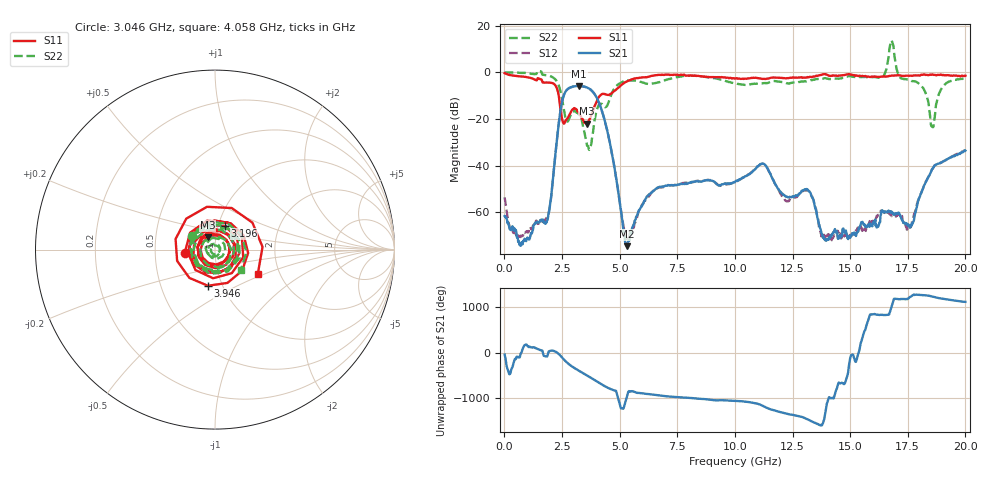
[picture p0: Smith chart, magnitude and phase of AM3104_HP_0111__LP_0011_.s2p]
!Created with skrf (http://scikit-rf.org).
# Hz S RI R 50.0
!freq ReS11 ImS11 ReS21 ImS21 ReS12 ImS12 ReS22 ImS22
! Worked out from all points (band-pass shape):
!   1601 points, 10 MHz to 20 GHz, reference 50 ohm
!   highest |S21| = -5.81 dB at 3.246 GHz (marker M1); lowest = -74.5 dB at 5.332 GHz (marker M2)
!   |S21| within 3 dB of the highest: 2.622 GHz to 3.878 GHz (1.256 GHz wide, 38.6 % of centre)
!   lowest |S11| = -22.1 dB at 3.571 GHz (marker M3), VSWR 1.17, Z = 45.7 + j6.24 ohm
!   |S11| at or under -10 dB: 2.358 GHz to 4.148 GHz (1.79 GHz wide, 55 % of centre)
!   |S22| runs from -33.3 to 13.7 dB; largest |S21 - S12| = 0.027
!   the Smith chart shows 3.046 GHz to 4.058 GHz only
!   S11 on the Smith chart (normalised r, x): 3.046 GHz: 0.71, -0.03; 3.196 GHz: 1.07, +0.29; 3.946 GHz: 0.85, -0.36; 4.058 GHz: 1.55, -0.45
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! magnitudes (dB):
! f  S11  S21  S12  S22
! 10 MHz  -0.4  -61.7  -53.5  0.0
! 572.2 MHz  -1.6  -70.8  -70.1  -0.1
! 1.822 GHz  -4.4  -64.1  -62.4  -1.2
! 2.496 GHz  -19.7  -12.8  -12.9  -11.1
! 3.046 GHz  -15.4  -6.0  -6.0  -16.5
! 3.196 GHz  -16.9  -5.8  -5.9  -17.5
! 3.246 GHz  -17.7  -5.8  -5.9  -18.3
! 3.346 GHz  -19.4  -5.9  -6.0  -20.0
! 3.571 GHz  -22.1  -6.4  -6.5  -30.4
! 3.946 GHz  -13.8  -9.8  -9.8  -18.8
! 4.058 GHz  -11.2  -11.9  -12.0  -14.7
! 5.332 GHz  -3.8  -74.5  -70.9  -3.3
! 6.682 GHz  -1.1  -49.3  -49.4  -4.3
! 10.01 GHz  -2.7  -47.1  -47.1  -4.8
! 11.2 GHz  -2.8  -39.1  -39.2  -4.7
! 13.34 GHz  -2.0  -53.4  -53.1  -3.3
! 13.98 GHz  -1.0  -71.8  -69.9  -2.6
! 16.68 GHz  -1.6  -59.4  -60.2  7.2
! 17.65 GHz  -1.4  -65.3  -65.7  -3.7
! 18.56 GHz  -0.9  -41.4  -41.5  -23.4
! 19.01 GHz  -1.2  -38.4  -38.3  -6.3
! 20 GHz  -1.4  -33.6  -33.5  -2.5
